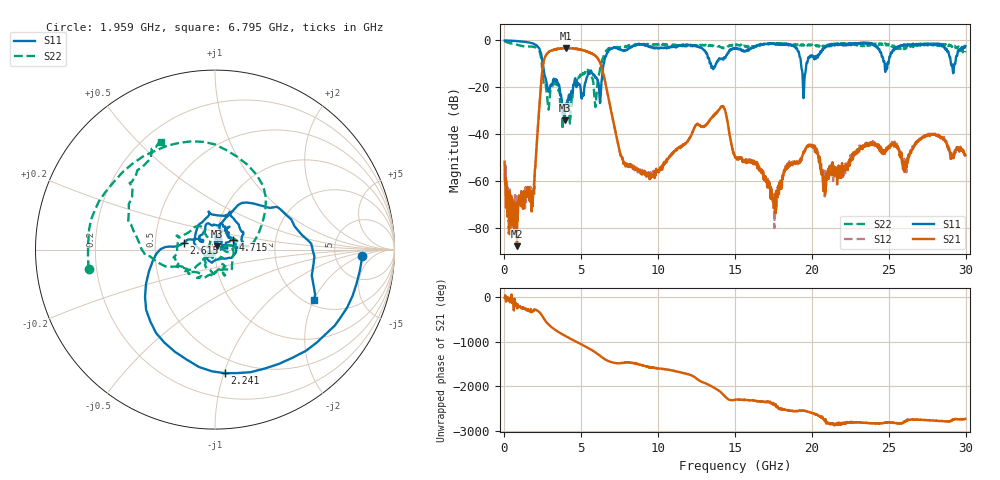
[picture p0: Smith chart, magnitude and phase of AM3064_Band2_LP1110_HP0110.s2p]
# Hz S DB R 50.0
!freq dBS11 angS11 dBS21 angS21 dBS12 angS12 dBS22 angS22
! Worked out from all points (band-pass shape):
!   1600 points, 10 MHz to 29.98 GHz, reference 50 ohm
!   highest |S21| = -3.21 dB at 4.002 GHz (marker M1); lowest = -87.9 dB at 816 MHz (marker M2)
!   |S21| within 3 dB of the highest: 2.717 GHz to 5.833 GHz (3.117 GHz wide, 72.9 % of centre)
!   lowest |S11| = -34.2 dB at 3.909 GHz (marker M3), VSWR 1.04, Z = 50.9 + j1.76 ohm
!   |S11| at or under -10 dB: 2.492 GHz to 6.458 GHz (3.965 GHz wide, 88.6 % of centre); 13.43 GHz to 13.77 GHz (343 MHz wide, 2.52 % of centre); 19.29 GHz to 19.64 GHz (349.5 MHz wide, 1.8 % of centre)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
!   |S22| runs from -37.9 to -0.3 dB; largest |S21 - S12| = 0.023
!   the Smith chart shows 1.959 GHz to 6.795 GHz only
!   S11 on the Smith chart (normalised r, x): 1.959 GHz: 9.66, -2.28; 2.241 GHz: 0.38, -1.01; 2.615 GHz: 0.70, +0.05; 4.715 GHz: 1.22, +0.14; 6.795 GHz: 2.20, -2.01
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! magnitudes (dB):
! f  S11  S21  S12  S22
! 10 MHz  0.0  -51.8  -57.0  -0.3
! 816 MHz  -0.3  -87.9  -75.0  -1.8
! 1.959 GHz  -1.7  -58.1  -57.8  -2.9
! 2.241 GHz  -3.2  -31.1  -31.1  -4.2
! 2.615 GHz  -15.0  -7.6  -7.5  -19.1
! 3.909 GHz  -34.2  -3.5  -3.2  -30.3
! 4.002 GHz  -27.0  -3.2  -3.4  -27.2
! 4.715 GHz  -18.7  -3.8  -3.6  -17.2
! 5.015 GHz  -24.7  -4.0  -4.0  -16.0
! 5.933 GHz  -16.1  -6.7  -6.8  -27.5
! 6.795 GHz  -4.2  -25.6  -25.6  -3.4
! 7.845 GHz  -4.5  -52.5  -52.5  -2.7
! 10 GHz  -3.4  -55.7  -55.6  -1.7
! 14.14 GHz  -7.8  -28.2  -28.3  -2.9
! 15 GHz  -3.2  -50.1  -49.2  -2.0
! 17.55 GHz  -1.6  -70.2  -80.2  -1.5
! 19 GHz  -3.4  -52.2  -51.6  -2.1
! 19.47 GHz  -24.0  -47.3  -47.5  -2.2
! 19.99 GHz  -6.3  -44.9  -45.4  -1.8
! 20.85 GHz  -3.0  -66.0  -58.3  -2.4
! 25 GHz  -9.0  -45.0  -45.5  -1.6
! 29.98 GHz  -2.4  -49.0  -48.9  -4.6
